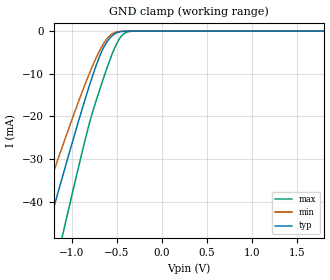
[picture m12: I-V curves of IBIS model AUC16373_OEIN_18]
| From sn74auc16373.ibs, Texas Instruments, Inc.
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[Model]   AUC16373_OEIN_18
Model_type  Input
Vinl=0.5775
Vinh=1.2675
| variable   typ   min   max
C_comp   2.51pF   2.05pF   2.88pF
[Temperature Range]   40   100   -40
| Ambient temperature   25   85   -40
[Voltage range]   1.8   1.65   1.95
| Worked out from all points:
|   GND clamp passes 1 mA (typ) near -0.55 V on its own axis
[GND Clamp]
| AUC16373_OEIN_18
|   Voltage   I(typ)   I(min)   I(max)
-3.6V     -226.6mA   -190.3mA   -271.8mA
-1.435V   -59.19mA   -47.53mA   -78.05mA
-1.26V    -45.87mA   -36.57mA   -62.17mA
-1.105V   -34.25mA   -27.09mA   -48.1mA
-1.08V    -32.4mA    -25.59mA   -45.83mA
-810mV    -13.15mA   -10.23mA   -22.06mA
-685mV    -5.638mA   -4.364mA   -13.41mA
-565mV    -1.378mA   -858.8uA   -6.102mA
-490mV    -325.9uA   -162.9uA   -2.495mA
-425mV    -63.96uA   -31.11uA   -688.8uA
-300mV    -1.501uA   -1.001uA   -11.88uA
1.8V      203.2pA    298.4pA    235.5pA
